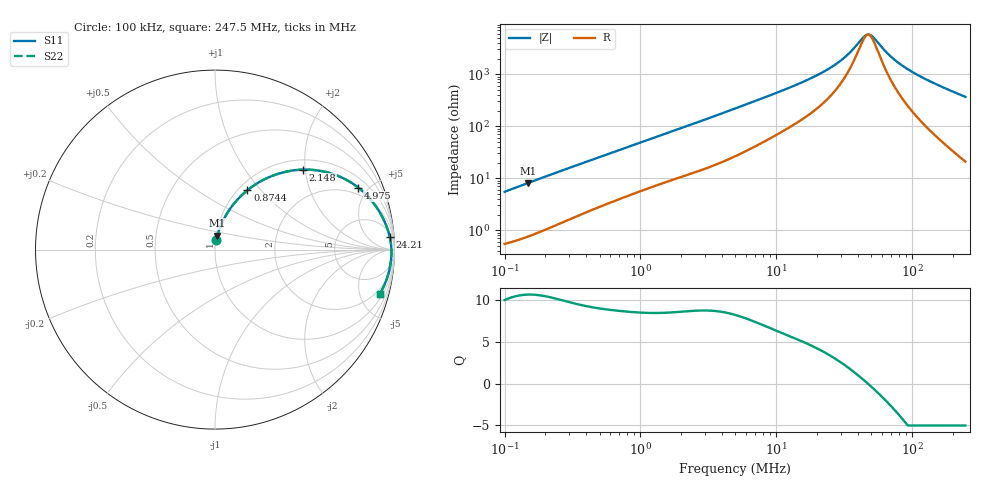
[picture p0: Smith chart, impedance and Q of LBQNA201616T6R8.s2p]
! LBQNA201616T6R8  S-PARAMETER MODEL  ( General Type )
! Model Generated by TAIYO YUDEN Corporation (http://www.ty-top.com)
! Version 1.0
! TAIYO YUDEN Control No. 191025NI43SB-FBB
! Copyright(c) 2019 TAIYO YUDEN CO.,LTD. All Rights Reserved.
! Product Description (link to TY-COMPAS)
! https://ds.yuden.co.jp/TYCOMPAS/or/detail?pn=LBQNA201616T6R8M&u=M
! Products Name : Inductors
! Characteristics :
!  Inductance : 6.8 uH , SRF(min) : 38 MHz , DC Resistance(max) : 0.455 Ohm
!  Rated Current : Saturation :300 mA , Temp Rise : 330 mA (20 degC)
!  Case Size : 2.0 x 1.6 / 0.079 x 0.063 [mm/inch] , Thickness : 1.6 / 0.063 [mm/inch]
!  (Conditions: Temperature = 25 degC , DC Bias Current/Voltage = 0A / 0V)
! External Node Assignments :
!  1  o---GGG---o  2
! GND o---------o GND
! Frequency Range : 0.1MHz  -  247.502633MHz  [ 402 STEP ]
# MHz S RI R 50
! Freq[MHz].  S11 Real  S11 Imag  S21 Real  S21 Imag  S12 Real  S12 Imag  S22 Real  S22 Imag
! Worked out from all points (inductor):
!   401 points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, 100 kHz to 247.5 MHz, reference 50 ohm
!   read as one part in series: L = 8.63 uH near 104 kHz
!   highest Q = 10.7 at 147.8 kHz (marker M1), where L = 8.6 uH
!   self-resonance near 47.49 MHz
!   S11 on the Smith chart (normalised r, x): 100 kHz: 1.01, +0.11; 874.4 kHz: 1.10, +0.85; 2.148 MHz: 1.22, +1.94; 4.975 MHz: 1.53, +4.34; 24.21 MHz: 8, +24; 247.5 MHz: 1.42, -7.32
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0.1  0.00832 0.0537  0.9917 -0.0537  0.9917 -0.0537  0.00832 0.0537
0.147802  0.0136 0.0782  0.9864 -0.0782  0.9864 -0.0782  0.0136 0.0782
0.37019  0.0532 0.1774  0.9468 -0.1774  0.9468 -0.1774  0.0532 0.1774
0.591615  0.1053 0.2556  0.8947 -0.2556  0.8947 -0.2556  0.1053 0.2556
0.874417  0.1804 0.3307  0.8196 -0.3307  0.8196 -0.3307  0.1804 0.3307
1.370406  0.3135 0.4087  0.6865 -0.4087  0.6865 -0.4087  0.3135 0.4087
2.147732  0.4902 0.4456  0.5098 -0.4456  0.5098 -0.4456  0.4902 0.4456
3.112971  0.6435 0.4254  0.3565 -0.4254  0.3565 -0.4254  0.6435 0.4254
4.974964  0.7994 0.3444  0.2006 -0.3444  0.2006 -0.3444  0.7994 0.3444
8.766464  0.9064 0.2265  0.0936 -0.2265  0.0936 -0.2265  0.9064 0.2265
18.41681  0.9636 0.107  0.0364 -0.107  0.0364 -0.107  0.9636 0.107
24.20972  0.9732 0.0729  0.0268 -0.0729  0.0268 -0.0729  0.9732 0.0729
32.45257  0.9795 0.0399  0.0205 -0.0399  0.0205 -0.0399  0.9795 0.0399
43.50191  0.9826 0.0091  0.0174 -0.0091  0.0174 -0.0091  0.9826 0.0091
47.03749  0.983 0.000988  0.017 -0.000988  0.017 -0.000988  0.983 0.000988
48.91162  0.9832 -0.00308  0.0168 0.00308  0.0168 0.00308  0.9832 -0.00308
51.86374  0.9833 -0.0092  0.0167 0.0092  0.0167 0.0092  0.9833 -0.0092
68.1772  0.9825 -0.0386  0.0175 0.0386  0.0175 0.0386  0.9825 -0.0386
84.52061  0.9803 -0.0636  0.0197 0.0636  0.0197 0.0636  0.9803 -0.0636
111.1061  0.9745 -0.0995  0.0255 0.0995  0.0255 0.0995  0.9745 -0.0995
164.2165  0.9574 -0.1621  0.0426 0.1621  0.0426 0.1621  0.9574 -0.1621
247.5026  0.9186 -0.2465  0.0814 0.2465  0.0814 0.2465  0.9186 -0.2465
